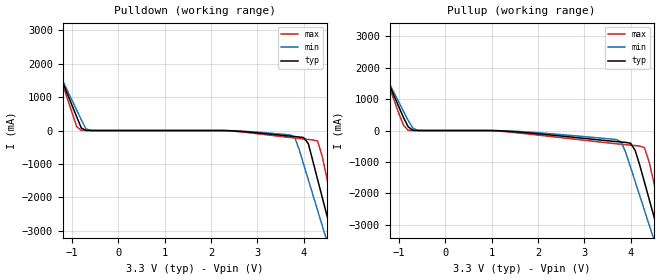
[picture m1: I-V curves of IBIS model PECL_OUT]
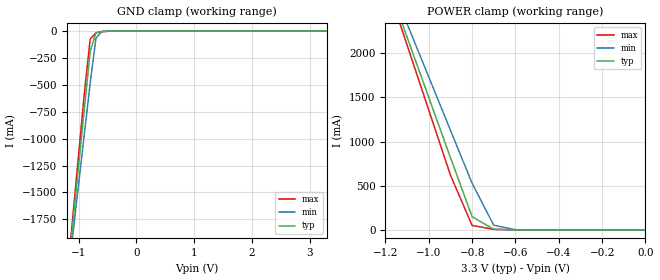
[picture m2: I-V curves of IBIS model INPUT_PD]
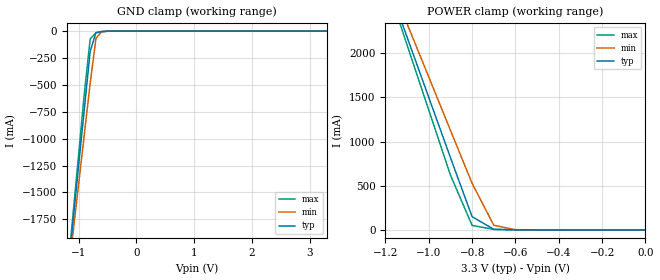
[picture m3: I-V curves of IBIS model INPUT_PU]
|   This file is an IBIS representation of the   |
|   Integrated Circuit Systems, Inc.   |
|   ICS87993I   |
|   LVPECL Output Frequency Synthesizer   |
[IBIS Ver]   3.2
[File name]   87993i.ibs
[File Rev]   1.0
[Date]   Jul 31 2003 | Last Modified
|   Jul 31 2003 | Generated
|   Created By Albert
[Source] Originated at Integrated Circuit Systems, Inc.
[Disclaimer]
(C) Copyright Integrated Circuit Systems, Inc. 1997
   All rights reserved
ICS hereby grants the user of this IBIS model a non-exclusive,
nontransferable license to use this IBIS model under the following terms.
Before using this IBIS model, the user should read this license.
If the user does not accept these terms,  the IBIS model should be
returned to ICS within 30 days.
   The user is granted this license only to use the IBIS model and
is not granted rights to sell, load, rent, lease or license the IBIS
model in whole or in part, or in modified form to anyone other than
user. User may modify the IBIS model to suit its specific
applications but rights to derivative works and such modifications
shall belong to ICS.
   This IBIS model is provided on an "AS IS" basis and ICS makes
absolutely no warranty with respect to the information contained
herein. ICS DISCLAIMS AND CUSTOMER WAIVES ALL WARRANTIES, EXPRESS
OR IMPLIED, INCLUDING WARRANTIES OF MERCHANTABILITY OR FITNESS FOR
A PARTICULAR PURPOSE. The entire risk as to quality and performance
is with the Customer. ACCORDINGLY, IN NO EVENT SHALL THE COMPANY BE
LIABLE FOR ANY DAMAGES, WHETHER IN CONTRACT OR TORT,INCLUDING ANY
LOST PROFITS OR OTHER INCIDENTAL, CONSEQUENTIAL, EXEMPLARY, OR
PUNITIVE DAMAGES ARISING OUT OF THE USE OR APPLICATION OF THE IBIS
model provided in this package. Further, ICS reserves the right to
make changes without notice to any product herein to improve
reliability, function, or design. ICS does not convey any license
under patent rights or any other intellectual property rights,
including those of third parties.
   ICS is not obligated to provide maintenance or support
for the licensed IBIS model.
[Copyright]   Copyright 2003 by Integrated Circuit Systems, Inc.
[Component]   ICS87993I
[Manufacturer] Integrated Circuit Systems, Inc.
[Package]
|   typ   min   max
R_pkg   8.5m   7.8m   9.2m
L_pkg   0.85nH   0.799nH   0.904nH
C_pkg   0.206pF   0.202pF   0.211pF
[Pin] signal_name   model_name
1   nMR   INPUT_PU
2   nALARM_RESET   INPUT_PU
3   CLK0   INPUT_PD
4   nCLK0   INPUT_PU
5   SEL_CLK   INPUT_PD
6   CLK1   INPUT_PD
7   nCLK1   INPUT_PU
8   VEE   GND
9   VEE   GND
10   EXT_FB   INPUT_PD
11   nEXT_FB   INPUT_PU
12   VEE   GND
|13   CLK_SELECTED
|14   INP1BAD
|15   INP0BAD
16   VCC   POWER
17   VCC   POWER
18   nQB2   PECL_OUT
19   QB2   PECL_OUT
20   nQB1   PECL_OUT
21   QB1   PECL_OUT
22   nQB0   PECL_OUT
23   QB0   PECL_OUT
24   VCC   POWER
25   nQA1   PECL_OUT
26   QA1   PECL_OUT
27   nQA0   PECL_OUT
28   QA0   PECL_OUT
29   VCC   POWER
30   VCCA   POWER
31   MAN_OVERRIDE   INPUT_PD
32   PLL_SEL   INPUT_PU
[Diff Pin]  inv_pin  vdiff tdelay_typ tdelay_min  tdelay_max
18   19   NA   0  0  0
20   21   NA   0  0  0
22   23   NA   0  0  0
25   26   NA   0  0  0
27   28   NA   0  0  0
| Models and submodels in the file (3): PECL_OUT (Output_ECL), INPUT_PD (Input), INPUT_PU (Input)
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[Model]   PECL_OUT
Model_type  Output_ECL
Polarity   Non-Inverting
|Variable   typ   min   max
C_comp   2p   1.5p   2.5p
|Variable   typ   min   max
[Temperature Range]   25   -40   85
|vddo
[Voltage Range]   3.3   3.135   3.465
|  Voltage   I(typ)   I(min)   I(max)
[Pullup]
-3.3V     8.64A      7.62A      10.24A
-1.9V     3.831A     3.523A     4.325A
-1.7V     3.145A     2.94A      3.481A
-800mV    117.7mA    321.6mA    7.854mA
-600mV    578.7uA    5.037mA    444.5uA
3.7V      -353.7mA   -289.1mA   -423.5mA
4V        -404.8mA   -1.175A    -467.2mA
4.2V      -1.116A    -2.09A     -495.5mA
4.3V      -1.651A    -2.547A    -544.5mA
4.6V      -3.257A    -3.919A    -2.296A
4.8V      -4.328A    -4.834A    -3.608A
6.6V      -13.98A    -13.09A    -15.44A
[Pulldown]
-3.3V     8.64A      7.62A      10.24A
-1.8V     3.488A     3.231A     3.903A
-1.6V     2.802A     2.648A     3.06A
-800mV    75.12mA    321.5mA    5.806mA
-600mV    445.9uA    3.217mA    366.5uA
3.7V      -165.8mA   -130.3mA   -208.8mA
3.8V      -179.2mA   -184.5mA   -224.1mA
4.1V      -392.4mA   -1.472A    -268mA
4.3V      -1.463A    -2.386A    -314.3mA
4.6V      -3.069A    -3.756A    -2.085A
4.8V      -4.139A    -4.67A     -3.398A
6.6V      -13.86A    -12.95A    -15.33A
[Ramp]
|   typ   min   max
dV/dt_r   0.45V/0.37ns   0.45V/0.405ns   0.45V/0.27ns
dV/dt_f   0.45V/0.37ns   0.45V/0.405ns   0.45V/0.27ns
R_load =   50.0000
[Model]   INPUT_PD
Model_type   Input
Polarity   Non-Inverting
Vinl = 1.4V
Vinh = 1.85V
|   typ   min   max
C_comp   2pF   1.5pF   2.5pF
|   typ   min   max
[Voltage range]  3.3V   3.15V   3.45V
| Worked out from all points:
|   GND clamp passes 1 mA (typ) near -0.51 V on its own axis
|   POWER clamp passes 1 mA (typ) near -0.60 V on its own axis
[GND_clamp]
|Voltage   I(typ)   I(min)   I(max)
-3.3V     -13.52A    -12.28A    -14.38A
-1.2V     -2.314A    -2.362A    -2.296A
-1.1V     -1.782A    -1.891A    -1.721A
-1V       -1.25A     -1.422A    -1.146A
-900mV    -718.5mA   -952.6mA   -572.1mA
-800mV    -188.2mA   -484.5mA   -72.95mA
-700mV    -13.66mA   -66.68mA   -15.82mA
-600mV    -3.044mA   -4.415mA   -6.968mA
-500mV    -658.9uA   -400.5uA   -2.169mA
3.3V      64.58uA    64.62uA    64.6uA
[POWER_clamp]
|Voltage   I(typ)   I(min)   I(max)
-3.3V     17.27A     15.67A     18.38A
-1.2V     2.866A     2.938A     2.832A
-1.1V     2.183A     2.334A     2.094A
-1V       1.501A     1.732A     1.358A
-900mV    819.8mA    1.13A      621.9mA
-800mV    150.3mA    528.4mA    51.58mA
-700mV    7.809mA    53.45mA    6.607mA
-600mV    968.4uA    3.161mA    1.955mA
0V        64.58uA    61.35uA    67.83uA
[Model]   INPUT_PU
Model_type   Input
Polarity   Non-Inverting
Vinl = 1.4V
Vinh = 1.85V
|   typ   min   max
C_comp   2pF   1.5pF   2.5pF
|   typ   min   max
[Voltage range]  3.3V   3.15V   3.45V
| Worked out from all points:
|   GND clamp passes 1 mA (typ) near -0.51 V on its own axis
|   POWER clamp passes 1 mA (typ) near -0.60 V on its own axis
[GND_clamp]
|Voltage   I(typ)   I(min)   I(max)
-3.3V     -13.52A    -12.28A    -14.38A
-1.2V     -2.314A    -2.362A    -2.296A
-1.1V     -1.782A    -1.891A    -1.721A
-1V       -1.25A     -1.422A    -1.146A
-900mV    -718.6mA   -952.7mA   -572.2mA
-800mV    -188.2mA   -484.6mA   -73.02mA
-700mV    -13.72mA   -66.74mA   -15.89mA
-600mV    -3.109mA   -4.477mA   -7.036mA
-500mV    -723.5uA   -462.1uA   -2.236mA
3.3V      3.748nA    2.972uA    -2.918uA
[POWER_clamp]
|Voltage   I(typ)   I(min)   I(max)
-3.3V     17.27A     15.67A     18.38A
-1.2V     2.866A     2.938A     2.832A
-1.1V     2.183A     2.334A     2.094A
-1V       1.501A     1.732A     1.358A
-900mV    819.7mA    1.129A     621.8mA
-800mV    150.2mA    528.4mA    51.51mA
-700mV    7.744mA    53.39mA    6.54mA
-600mV    903.9uA    3.099mA    1.887mA
0V        3.748nA    2.31nA     19.96nA
